|Texas Instruments Incorporated
|tmux5508,  1 data line 8:1 Mux
[IBIS Ver]   4.1
[File name]   tmux5508.ibs
[Date]   06/29/26
[File Rev]   1.0
[Source]
| Texas Instruments Incorporated.
| ASC-INT-MUX
| 12500 TI Blvd
| Dallas, TX - 75243
[Notes]   Revision History:
| Rev 1.0: 06/29/26
| - Initial version of the model
| - Model generated from simulations in SPECTRE
| - C_comp although listed in numerical order of value are
|   obtained from varying PVT conditions. For PVT conditions for
|   each specific value refer the buffer description under
|   respective [Model]. IBIS model user is responsible for using
|   appropriate C_comp to simulate for Signal Integrity.
[Disclaimer]
| This model is designed as an aid for customers of Texas Instruments.
| TI and its licensors and suppliers make no warranties, either expressed
| or implied, with respect to this  model, including the warranties of
| merchantability or fitness for a particular purpose. The model is
| provided solely on an "as is" basis. The entire risk as to its quality
| and performance is with the customer.
| This model is subject to change without notice. Texas Instruments
| Incorporated is not responsible for updating this model.
[Copyright]
(C) Copyright 2026 Texas Instruments Incorporated.All rights reserved.
|  Component TMUX5508D 16-pin - D package
|  Part # TMUX5508D
[Component]   TMUX5508D
[Manufacturer]  TI
[Package]
|   typ   min   max
R_pkg   0.075   NA   NA
L_pkg   1nH   NA   NA
C_pkg   0.25pF   NA   NA
[Pin]   signal_name   model_name
   1   A0   inbuf
   2   EN   inbuf
   3   VSS   power
   4   S1   sterm
   5   S2   sterm
   6   S3   sterm
   7   S4   sterm
   8   D   dterm
   9   S8   sterm
   10   S7   sterm
   11   S6   sterm
   12   S5   sterm
   13   VDD   power
   14   GND   gnd
   15   A2   inbuf
   16   A1   inbuf
[Series Switch Groups]
On 1 /
On 2 /
On 3 /
On 4 /
On 5 /
On 6 /
On 7 /
On 8 /
Off 1 /
[Series Pin Mapping]  pin_2 model_name function_table_group
   8   4   switch_dual_20   1
   8   5   switch_dual_20   1
   8   6   switch_dual_20   1
   8   7   switch_dual_20   1
   8   9   switch_dual_20   1
   8  10   switch_dual_20   1
   8  11   switch_dual_20   1
   8  12   switch_dual_20   1
|   8   4   switch_dual_15   1
|   8   5   switch_dual_15   1
|   8   6   switch_dual_15   1
|   8   7   switch_dual_15   1
|   8   9   switch_dual_15   1
|   8  10   switch_dual_15   1
|   8  11   switch_dual_15   1
|   8  12   switch_dual_15   1
|   8   4   switch_40   1
|   8   5   switch_40   1
|   8   6   switch_40   1
|   8   7   switch_40   1
|   8   9   switch_40   1
|   8  10   switch_40   1
|   8  11   switch_40   1
|   8  12   switch_40   1
|   8   4   switch_12   1
|   8   5   switch_12   1
|   8   6   switch_12   1
|   8   7   switch_12   1
|   8   9   switch_12   1
|   8  10   switch_12   1
|   8  11   switch_12   1
|   8  12   switch_12   1
|   8   4   switch_5   1
|   8   5   switch_5   1
|   8   6   switch_5   1
|   8   7   switch_5   1
|   8   9   switch_5   1
|   8  10   switch_5   1
|   8  11   switch_5   1
|   8  12   switch_5   1
|  Component TMUX5508PW 16-pin - PW package
|  Part # TMUX5508PW
[Component]   TMUX5508PW
[Manufacturer]  TI
[Package]
|   typ   min   max
R_pkg   0.075   NA   NA
L_pkg   1nH   NA   NA
C_pkg   0.25pF   NA   NA
[Pin]   signal_name   model_name
   1   A0   inbuf
   2   EN   inbuf
   3   VSS   power
   4   S1   sterm
   5   S2   sterm
   6   S3   sterm
   7   S4   sterm
   8   D   dterm
   9   S8   sterm
   10   S7   sterm
   11   S6   sterm
   12   S5   sterm
   13   VDD   power
   14   GND   gnd
   15   A2   inbuf
   16   A1   inbuf
[Series Switch Groups]
On 1 /
On 2 /
On 3 /
On 4 /
On 5 /
On 6 /
On 7 /
On 8 /
Off 1 /
[Series Pin Mapping]  pin_2 model_name function_table_group
   8   4   switch_dual_20   1
   8   5   switch_dual_20   1
   8   6   switch_dual_20   1
   8   7   switch_dual_20   1
   8   9   switch_dual_20   1
   8  10   switch_dual_20   1
   8  11   switch_dual_20   1
   8  12   switch_dual_20   1
|   8   4   switch_dual_15   1
|   8   5   switch_dual_15   1
|   8   6   switch_dual_15   1
|   8   7   switch_dual_15   1
|   8   9   switch_dual_15   1
|   8  10   switch_dual_15   1
|   8  11   switch_dual_15   1
|   8  12   switch_dual_15   1
|   8   4   switch_40   1
|   8   5   switch_40   1
|   8   6   switch_40   1
|   8   7   switch_40   1
|   8   9   switch_40   1
|   8  10   switch_40   1
|   8  11   switch_40   1
|   8  12   switch_40   1
|   8   4   switch_12   1
|   8   5   switch_12   1
|   8   6   switch_12   1
|   8   7   switch_12   1
|   8   9   switch_12   1
|   8  10   switch_12   1
|   8  11   switch_12   1
|   8  12   switch_12   1
|   8   4   switch_5   1
|   8   5   switch_5   1
|   8   6   switch_5   1
|   8   7   switch_5   1
|   8   9   switch_5   1
|   8  10   switch_5   1
|   8  11   switch_5   1
|   8  12   switch_5   1
|  Component TMUX5508RSV 16-pin - RSV package
|  Part # TMUX5508RSV
[Component]   TMUX5508RSV
[Manufacturer]  TI
[Package]
|   typ   min   max
R_pkg   0.075   NA   NA
L_pkg   1nH   NA   NA
C_pkg   0.25pF   NA   NA
[Pin]   signal_name   model_name
   1   A0   inbuf
   2   EN   inbuf
   3   VSS   power
   4   S1   sterm
   5   S2   sterm
   6   S3   sterm
   7   S4   sterm
   8   D   dterm
   9   S8   sterm
   10   S7   sterm
   11   S6   sterm
   12   S5   sterm
   13   VDD   power
   14   GND   gnd
   15   A2   inbuf
   16   A1   inbuf
[Series Switch Groups]
On 1 /
On 2 /
On 3 /
On 4 /
On 5 /
On 6 /
On 7 /
On 8 /
Off 1 /
[Series Pin Mapping]  pin_2 model_name function_table_group
   8   4   switch_dual_20   1
   8   5   switch_dual_20   1
   8   6   switch_dual_20   1
   8   7   switch_dual_20   1
   8   9   switch_dual_20   1
   8  10   switch_dual_20   1
   8  11   switch_dual_20   1
   8  12   switch_dual_20   1
|   8   4   switch_dual_15   1
|   8   5   switch_dual_15   1
|   8   6   switch_dual_15   1
|   8   7   switch_dual_15   1
|   8   9   switch_dual_15   1
|   8  10   switch_dual_15   1
|   8  11   switch_dual_15   1
|   8  12   switch_dual_15   1
|   8   4   switch_40   1
|   8   5   switch_40   1
|   8   6   switch_40   1
|   8   7   switch_40   1
|   8   9   switch_40   1
|   8  10   switch_40   1
|   8  11   switch_40   1
|   8  12   switch_40   1
|   8   4   switch_12   1
|   8   5   switch_12   1
|   8   6   switch_12   1
|   8   7   switch_12   1
|   8   9   switch_12   1
|   8  10   switch_12   1
|   8  11   switch_12   1
|   8  12   switch_12   1
|   8   4   switch_5   1
|   8   5   switch_5   1
|   8   6   switch_5   1
|   8   7   switch_5   1
|   8   9   switch_5   1
|   8  10   switch_5   1
|   8  11   switch_5   1
|   8  12   switch_5   1
[Model Selector] dterm
dterm_dual_20 Use for operation at +/-20V
dterm_dual_15 Use for operation at +/-15V
dterm_40 Use for operation at 40V
dterm_12 Use for operation at 12V
dterm_5 Use for operation at 5V
[Model Selector] sterm
sterm_dual_20 Use for operation at +/-20V
sterm_dual_15 Use for operation at +/-15V
sterm_40 Use for operation at 40V
sterm_12 Use for operation at 12V
sterm_5 Use for operation at 5V
[Model Selector] inbuf
inbuf_dual_20 Use for operation at +/-20V
inbuf_dual_15 Use for operation at +/-15V
inbuf_40 Use for operation at 40V
inbuf_12 Use for operation at 12V
inbuf_5 Use for operation at 5V
| switch_dual_20
[Model]   switch_dual_20
Model_type   Series_switch
|   typ   min   max
C_comp   2.533030e-12   NA   NA
[Voltage Range]   20   NA   NA
[Power Clamp Reference]   20   NA   NA
[Temperature Range]   27   NA   NA
[On]
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[Off]
|   typ   min   max
[R Series]   10G   NA   NA
| switch_dual_15
[Model]   switch_dual_15
Model_type   Series_switch
|   typ   min   max
C_comp   2.533030e-12   NA   NA
[Voltage Range]   15   NA   NA
[Power Clamp Reference]   15   NA   NA
[Temperature Range]   27   NA   NA
[On]
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[Off]
|   typ   min   max
[R Series]   10G   NA   NA
| switch_40
[Model]   switch_40
Model_type   Series_switch
|   typ   min   max
C_comp   2.533030e-12   NA   NA
[Voltage Range]   40   NA   NA
[Power Clamp Reference]   40   NA   NA
[Temperature Range]   27   NA   NA
[On]
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[Off]
|   typ   min   max
[R Series]   10G   NA   NA
| switch_12
[Model]   switch_12
Model_type   Series_switch
|   typ   min   max
C_comp   2.533030e-12   NA   NA
[Voltage Range]   12   NA   NA
[Power Clamp Reference]   12   NA   NA
[Temperature Range]   27   NA   NA
[On]
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[Off]
|   typ   min   max
[R Series]   10G   NA   NA
| switch_5
[Model]   switch_5
Model_type   Series_switch
|   typ   min   max
C_comp   2.533030e-12   NA   NA
[Voltage Range]   5   NA   NA
[Power Clamp Reference]   5   NA   NA
[Temperature Range]   27   NA   NA
[On]
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[Off]
|   typ   min   max
[R Series]   10G   NA   NA
| Models and submodels in the file (20): dterm_dual_20 (Terminator), dterm_dual_15 (Terminator), dterm_40 (Terminator), dterm_12 (Terminator), dterm_5 (Terminator), switch_dual_20 (Series_switch), switch_dual_15 (Series_switch), switch_40 (Series_switch), switch_12 (Series_switch), switch_5 (Series_switch), sterm_dual_20 (Terminator), sterm_dual_15 (Terminator), sterm_40 (Terminator), sterm_12 (Terminator), sterm_5 (Terminator), inbuf_dual_20 (Input), inbuf_dual_15 (Input), inbuf_40 (Input), inbuf_12 (Input), inbuf_5 (Input)
